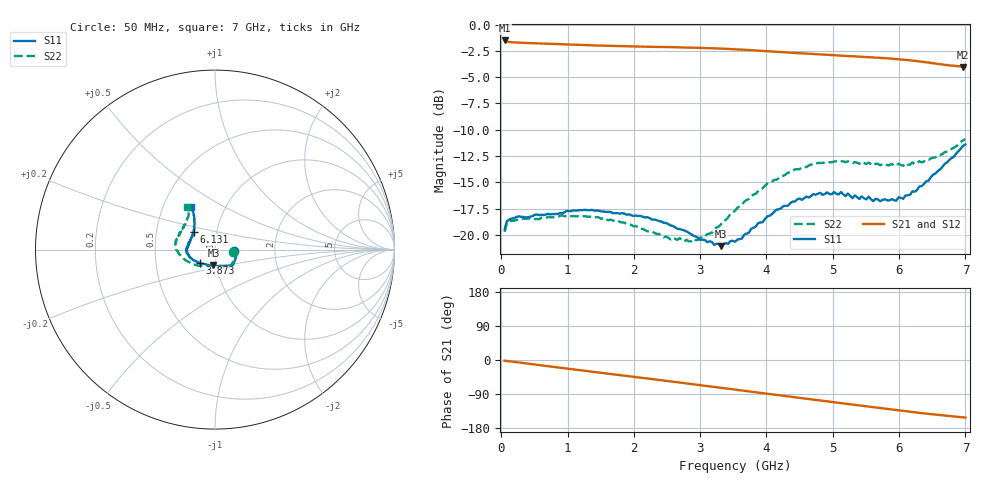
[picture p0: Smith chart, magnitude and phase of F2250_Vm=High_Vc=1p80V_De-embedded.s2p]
! Integrated Device Technology
! Corporate Headquarters
! 6024 Silver Creek Valley Road
! San Jose, CA 95138  USA
! Phone:  1-408-284-8200
! Toll Free:  1-800-223-1366
! Webpage:  http://www.idt.com/
! Timing and RF Division
! 515 Groton Road, Suite 102
! Westford, MA 01886-6024
! Device:  F2250
! Description: Voltage Variable RF Attenuator
! Frequency:  50.0 -  6000.00 MHz
! Package:  3x3 mm Thin QFN Plastic Package: 16 pin
! Ports:  2 RF, 3 DC
!  Pin  1  = GND
!  Pin  2  = NC
!  Pin  3  = RF1  = Port 1
!  Pin  4  = NC
!  Pin  5  = GND
!  Pin  6  = GND
!  Pin  7  = GND
!  Pin  8  = GND
!  Pin  9  = NC
!  Pin 10  = RF2  = Port 2
!  Pin 11  = NC
!  Pin 12  = GND
!  Pin 13  = GND
!  Pin 14  = VCNTRL
!  Pin 15  = VDD
!  Pin 16  = VMODE
! Vcntrl:  1.800 Volts
! Vmode:  +3.300 Volts
! Vdd:  +3.30  Volts
! Current:  1.323 mA
! Data:  The device was measured on a the F2250 evaluation board which has
!  individual transmission lines to the RF pins.  Data was collected
!  using a calibrated network analyzer.  The evaluation board was
!  de-embedded using a TRL calibration technique.
!  The reference plane is the edge of the package pin.
! Misc:  SN 10
!  Action Tracker AT0258
! Date Measured:  2014-11-26
! Date:  2015-10-15  MJV
! Note:
!  Integrated Device Technology supplies this data as a sample of measured
!  data at the package pin for this product.  Your particular data for this
!  product may vary.
!  Data was taken at 25 degrees C.
!  Integrated Device Technology reserves the right to change this data at anytime.
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# GHz S dB R 50
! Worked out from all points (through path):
!   201 points, 50 MHz to 7 GHz, reference 50 ohm
!   highest |S21| = -1.52 dB at 50 MHz (marker M1); lowest = -4.0 dB at 6.965 GHz (marker M2)
!   group delay of S21, straight-line fit = 61 ps
!   lowest |S11| = -21.1 dB at 3.317 GHz (marker M3), VSWR 1.19, Z = 48.4 - j8.59 ohm
!   |S11| at or under -10 dB: start of sweep to end of sweep
!   |S22| runs from -20.6 to -10.9 dB; largest |S21 - S12| = 0.0018
!   S11 on the Smith chart (normalised r, x): 50 MHz: 1.24, -0.02; 3.873 GHz: 0.83, -0.13; 6.131 GHz: 0.77, +0.16; 7 GHz: 0.69, +0.35
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0.05  -19.46 -5.1  -1.52 -1.9  -1.52 -1.9  -19.69 -6.4
0.08475  -18.68 -5.0  -1.62 -2.5  -1.62 -2.5  -18.87 -6.1
0.1195  -18.53 -5.7  -1.66 -3.3  -1.67 -3.3  -18.67 -6.2
0.745  -18.03 -27.1  -1.83 -17.2  -1.83 -17.2  -18.32 -32.6
1.2315  -17.63 -40.2  -1.95 -27.9  -1.95 -27.9  -18.20 -50.5
1.75275  -17.92 -47.2  -2.04 -39.0  -2.05 -39.1  -18.61 -61.4
2.37825  -18.67 -50.7  -2.13 -52.6  -2.14 -52.6  -19.89 -72.5
2.86475  -19.92 -63.2  -2.20 -63.4  -2.20 -63.4  -20.60 -94.8
3.1775  -20.67 -82.1  -2.26 -70.4  -2.26 -70.5  -19.78 -116.2
3.3165  -21.06 -95.7  -2.29 -73.6  -2.29 -73.7  -18.96 -125.6
3.525  -20.64 -113.2  -2.35 -78.4  -2.36 -78.4  -17.69 -137.5
3.8725  -18.87 -138.2  -2.48 -86.2  -2.49 -86.2  -15.85 -154.9
4.4285  -16.81 -162.2  -2.71 -98.5  -2.71 -98.6  -13.75 -174.2
4.7065  -16.11 -171.2  -2.80 -104.7  -2.81 -104.7  -13.33 179.2
5.1235  -15.91 178.1  -2.96 -113.8  -2.96 -113.9  -13.00 169.3
5.29725  -16.50 172.4  -3.01 -117.6  -3.01 -117.6  -13.16 165.8
5.332  -16.23 171.1  -3.03 -118.4  -3.02 -118.4  -13.06 164.9
5.85325  -16.72 152.7  -3.23 -129.7  -3.23 -129.8  -13.37 151.1
6.13125  -16.23 140.5  -3.38 -135.7  -3.39 -135.8  -13.32 143.6
6.54825  -14.15 126.5  -3.70 -144.4  -3.70 -144.5  -12.62 130.0
6.96525  -11.52 119.8  -4.02 -151.3  -4.02 -151.4  -11.01 123.9
7  -11.40 119.4  -4.02 -151.8  -4.03 -151.9  -10.88 123.1
